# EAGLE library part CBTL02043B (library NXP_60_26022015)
AAL Eindhoven MK
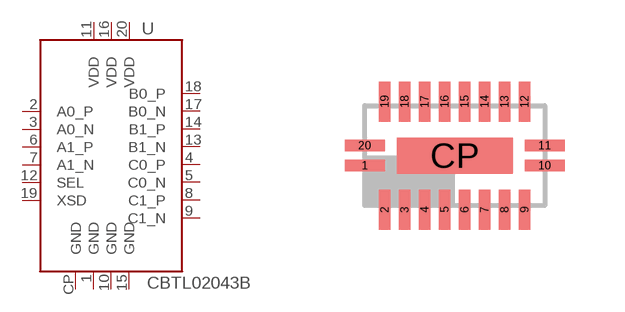
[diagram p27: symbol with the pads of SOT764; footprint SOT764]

Designator prefix U

## CBTL02043BBQ  [SOT764]
1  GND
2  A0_P
3  A0_N
4  C0_P
5  C0_N
6  A1_P
7  A1_N
8  C1_P
9  C1_N
10  GND
11  VDD
12  SEL  in
13  B1_N
14  B1_P
15  GND
16  VDD
17  B0_N
18  B0_P
19  XSD  in
20  VDD
CP  GND

## Footprint SOT764 (pad centres in mm)
SOT764 DHVQFN20: plastic dual in-line compatible thermal enhanced very thin quad flat package; no leads; 20 terminals; body 2.5 x 4.5 x 0.85 mm JEDEC: MO-241 IEC: ---
smd 1 x 0.29: 1 -2.25,-0.25; 10 2.25,-0.25; 11 2.25,0.25; 20 -2.25,0.25
smd 0.29 x 1: 2 -1.75,-1.35; 3 -1.25,-1.35; 4 -0.75,-1.35; 5 -0.25,-1.35; 6 0.25,-1.35; 7 0.75,-1.35; 8 1.25,-1.35; 9 1.75,-1.35; 12 1.75,1.35; 13 1.25,1.35; 14 0.75,1.35; 15 0.25,1.35; 16 -0.25,1.35; 17 -0.75,1.35; 18 -1.25,1.35; 19 -1.75,1.35
smd 2.9 x 0.9: CP 0,0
